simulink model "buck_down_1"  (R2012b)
settings: Solver=ode45  StartTime=0.0  StopTime=10.0  RelTol=1e-3
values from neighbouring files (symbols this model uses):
  C = 100e-6    (= 0.0001)    [boost_up1.m]    (also in buck_boost1.m = 0.0002; buck_boost2.m = 0.0002; buck_down1.m; buck_down2.m)
  f0 = 0.2e5    (= 20000)    [boost_up1.m]    (also in buck_boost1.m; buck_boost2.m; buck_down1.m; buck_down2.m)
  L = 0.001    [boost_up1.m]    (also in buck_boost1.m; buck_boost2.m; buck_down1.m; buck_down2.m)
  R = 5    [boost_up1.m]    (also in buck_boost1.m; buck_boost2.m; buck_down1.m = 2*Rmax,; buck_down2.m = 0.1*Rmax,)
  Ui = 5    [boost_up1.m]    (also in buck_boost1.m; buck_boost2.m; buck_down1.m; buck_down2.m)

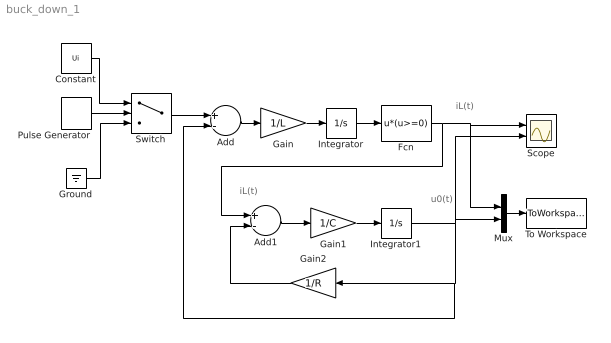
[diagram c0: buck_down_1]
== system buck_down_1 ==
  note: iL(t)
  note: u0(t)
  note: iL(t)
  Add : Sum  Inputs=+-
  Add1 : Sum  Inputs=+-
  Constant : Constant  Value=Ui
  Fcn : Fcn  Expr=u*(u>=0)
  Gain : Gain  Gain=1/L
  Gain1 : Gain  Gain=1/C
  Gain2 : Gain  Gain=1/R
  Ground : Ground
  Integrator : Integrator
  Integrator1 : Integrator
  Mux : Mux  Inputs=2
  Pulse Generator : DiscretePulseGenerator  PulseType=Time based  Period=1/f0  PulseWidth=50
  Scope : Scope  NumInputPorts=2
  Switch : Switch  Criteria=u2 > Threshold  Threshold=0.5  ZeroCross=off  SampleTime=0
  To Workspace : ToWorkspace  VariableName=y  SampleTime=-1  SaveFormat=Structure With Time
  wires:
  Pulse Generator/1 -> Switch/2
  Add/1 -> Gain/1
  Gain/1 -> Integrator/1
  Gain1/1 -> Integrator1/1
  Add1/1 -> Gain1/1
  Gain2/1 -> Add1/2
  Ground/1 -> Switch/3
  Constant/1 -> Switch/1
  Switch/1 -> Add/1
  Integrator1/1 -> Mux/2, Scope/2, Add/2, Gain2/1
  Integrator/1 -> Fcn/1
  Fcn/1 -> Add1/1, Mux/1, Scope/1
  Mux/1 -> To Workspace/1
